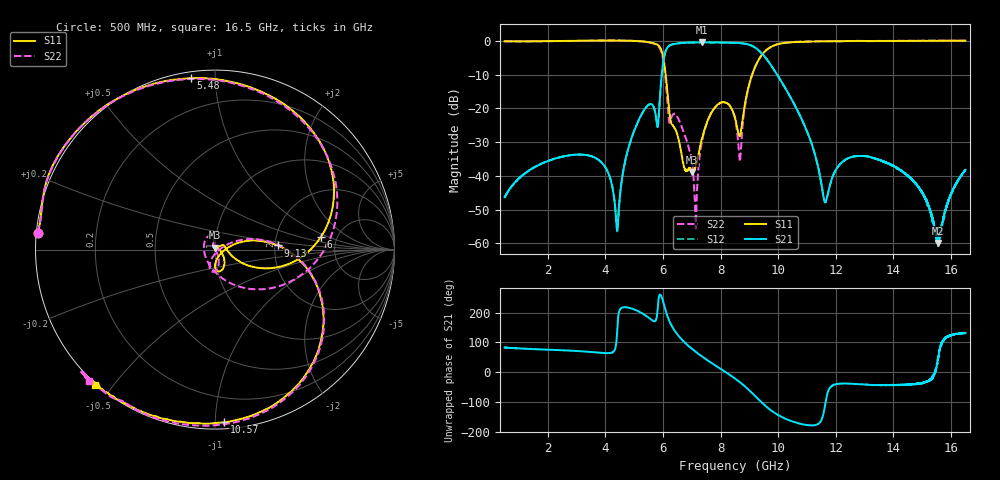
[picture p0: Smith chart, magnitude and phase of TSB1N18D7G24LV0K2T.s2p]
! TSB1N18D7G24LV0K2T  S-PARAMETER MODEL  ( General Type )
! Model Generated by TAIYO YUDEN Corporation (https://www.yuden.co.jp/en/)
! Version 1.0
! TAIYO YUDEN Control No. 20240527
! Copyright(c) 2024 TAIYO YUDEN CO.,LTD. All Rights Reserved.
! Products Name : Ceramic RF Devices
! Characteristics :
!  Passband freq : 6240-8250 MHz ( At Passband , Insertion Loss : 2.2dB , VSWR 2.0 )
!  Attenuation : 30 dB min at 617 to 4200MHz, 20 dB min at 4400to 5000MHz,  , Impedance : 50 Ohm
!  Case Size : 1.6 x 0.8 / 0.063 x 0.031 [mm/inch] , Thickness : 0.65/ 0.026 [mm/inch]
!  (Conditions: Temperature = 25 degC , DC Bias Current/Voltage = 0A / 0V)
! External Node Assignments :
!  1  o---|-------|---o  2
!  |  BPF  |
! GND o---|-------|---o GND
! Frequency Range : 500MHz  -  16.5GHz  [ 3201 STEP ]
# MHZ S RI R 50
! Freq[MHz].  S11 Real  S11 Imag  S21 Real  S21 Imag  S12 Real  S12 Imag  S22 Real  S22 Imag
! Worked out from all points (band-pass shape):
!   3201 points, 500 MHz to 16.5 GHz, reference 50 ohm
!   highest |S21| = -0.39 dB at 7.365 GHz (marker M1); lowest = -59.9 dB at 15.55 GHz (marker M2)
!   |S21| within 3 dB of the highest: 6.078 GHz to 9.402 GHz (3.324 GHz wide, 43 % of centre)
!   lowest |S11| = -39.0 dB at 7.015 GHz (marker M3), VSWR 1.02, Z = 50.1 + j1.12 ohm
!   |S11| at or under -10 dB: 6.093 GHz to 9.093 GHz (3 GHz wide, 39.5 % of centre)
!   |S22| runs from -55.7 to 0.1 dB; largest |S21 - S12| = 0.0027
!   S11 on the Smith chart (normalised r, x): 500 MHz: 0.00, +0.05; 5.48 GHz: 0.03, +0.87; 6 GHz: 3.74, +0.81; 9.13 GHz: 2.07, +0.11; 10.57 GHz: 0.04, -1.05; 16.5 GHz: -0.01, -0.45
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500  -0.9868 0.0924  0.000632 0.00478  0.000622 0.00474  -0.9854 0.0945
3170  -0.9444 0.3594  0.00704 0.0194  0.007 0.0195  -0.9436 0.3613
4025  -0.8871 0.5016  0.0056 0.0116  0.00557 0.0115  -0.8838 0.5023
4410  -0.8198 0.6021  -0.00124 0.000934  -0.00122 0.000945  -0.8177 0.6027
4790  -0.7002 0.7311  -0.0201 -0.0149  -0.02 -0.0148  -0.6978 0.7303
5480  -0.1363 0.955  -0.1115 -0.00901  -0.1112 -0.00885  -0.1186 0.9511
5835  0.5252 0.6821  -0.0345 -0.0506  -0.0345 -0.0505  0.5796 0.6019
6000  0.5898 0.0697  -0.2374 -0.3896  -0.237 -0.3894  0.5323 -0.0989
6270  0.0644 0.000682  -0.8294 0.2812  -0.8294 0.2813  -0.0611 0.0297
7015  0.00123 0.0112  0.2055 0.9288  0.2061 0.9269  -0.00561 0.0143
7150  0.0124 0.00847  0.3684 0.8793  0.3693 0.8777  0.00242 -0.000415
7365  0.0343 -0.0126  0.5887 0.7533  0.5879 0.7515  0.0156 -0.0305
8500  0.00303 -0.0734  0.8779 -0.337  0.8775 -0.3363  -0.025 -0.0662
8680  0.0357 -0.0183  0.7723 -0.5226  0.7716 -0.522  0.0151 -0.00848
9130  0.3498 0.0229  0.2435 -0.7961  0.2428 -0.7965  0.3465 0.0289
10570  0.0491 -0.9627  -0.1103 -0.0243  -0.1098 -0.0239  0.0827 -0.9678
11170  -0.2327 -0.954  -0.0293 -0.000972  -0.0293 -0.000914  -0.2059 -0.9693
11635  -0.3912 -0.9085  -0.00104 -0.00395  -0.00104 -0.00398  -0.3777 -0.9214
12375  -0.5579 -0.827  0.0141 -0.0108  0.014 -0.0109  -0.5614 -0.8292
13835  -0.6798 -0.7358  0.011 -0.0102  0.0111 -0.0103  -0.7307 -0.6889
15555  -0.6763 -0.7462  0.000702 0.000735  0.000712 0.000927  -0.724 -0.7072
16500  -0.6698 -0.7545  -0.00806 0.00926  -0.00799 0.00944  -0.7022 -0.7314
